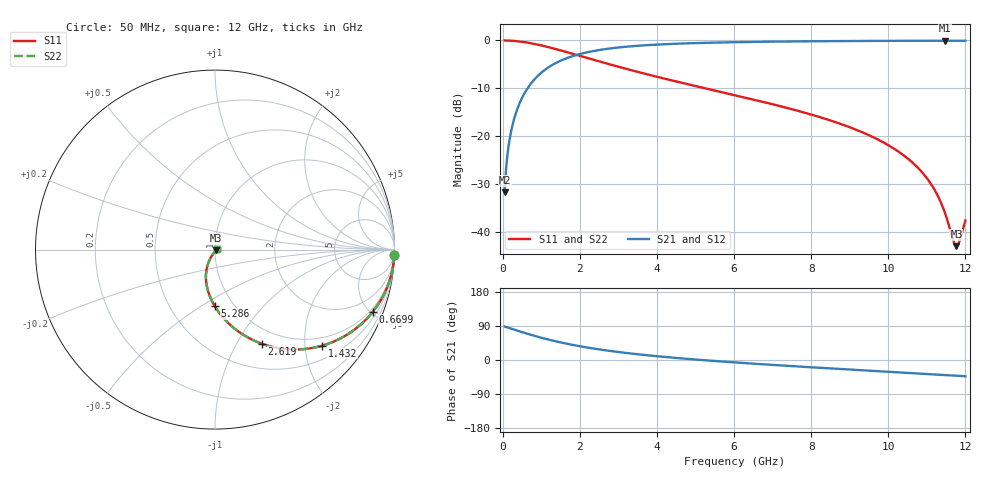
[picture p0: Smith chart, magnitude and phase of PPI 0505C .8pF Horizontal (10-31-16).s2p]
# MHz S MA R 50
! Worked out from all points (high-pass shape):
!   1601 points, 50 MHz to 12 GHz, reference 50 ohm
!   highest |S21| = -0.07 dB at 11.47 GHz (marker M1); lowest = -31.8 dB at 50 MHz (marker M2)
!   |S21| within 3 dB of the highest: 1.899 GHz to end of sweep
!   lowest |S11| = -43.0 dB at 11.77 GHz (marker M3), VSWR 1.01, Z = 50.5 - j0.486 ohm
!   |S11| at or under -10 dB: 5.255 GHz to end of sweep
!   |S22| runs from -43.0 to 0.0 dB; largest |S21 - S12| = 0
!   S11 on the Smith chart (normalised r, x): 50 MHz: 1, -69; 669.9 MHz: 0.79, -5.13; 1.432 GHz: 0.80, -2.38; 2.619 GHz: 0.80, -1.28; 5.286 GHz: 0.82, -0.57; 12 GHz: 1.03, +0.01
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50  0.9997 -1.7  0.02582 88.3  0.02582 88.3  0.9997 -1.7
162.0312  0.9965 -5.4  0.08342 84.6  0.08342 84.6  0.9965 -5.4
266.5938  0.9906 -8.8  0.1365 81.2  0.1365 81.2  0.9906 -8.8
438.375  0.9752 -14.4  0.221 75.6  0.221 75.6  0.9752 -14.4
669.9062  0.9447 -21.6  0.3273 68.4  0.3273 68.4  0.9447 -21.6
1006  0.8864 -31.2  0.4618 58.7  0.4618 58.7  0.8864 -31.2
1431.719  0.8018 -41.9  0.596 48.0  0.596 48.0  0.8018 -41.9
2044.156  0.6826 -54.3  0.7286 35.5  0.7286 35.5  0.6826 -54.3
2619.25  0.5861 -63.5  0.8076 26.2  0.8076 26.2  0.5861 -63.5
4038.312  0.414 -79.9  0.9068 9.6  0.9068 9.6  0.414 -79.9
5285.594  0.3142 -90.3  0.9452 -1.0  0.9452 -1.0  0.3142 -90.3
6025  0.2679 -95.5  0.9589 -6.4  0.9589 -6.4  0.2679 -95.5
8019.156  0.1675 -107.6  0.9803 -19.3  0.9803 -19.3  0.1675 -107.6
9154.406  0.1174 -113.4  0.9869 -26.1  0.9869 -26.1  0.1174 -113.4
10013.31  0.08006 -116.8  0.9901 -31.2  0.9901 -31.2  0.08006 -116.8
10917.03  0.04019 -117.0  0.992 -36.5  0.992 -36.5  0.04019 -117.0
11230.72  0.02621 -113.4  0.9922 -38.3  0.9922 -38.3  0.02621 -113.4
11469.72  0.01582 -103.8  0.9923 -39.7  0.9923 -39.7  0.01582 -103.8
11686.31  0.008127 -70.9  0.9922 -41.0  0.9922 -41.0  0.008127 -70.9
11768.47  0.007103 -42.6  0.9922 -41.5  0.9922 -41.5  0.007103 -42.6
11835.69  0.007777 -18.7  0.9921 -41.9  0.9921 -41.9  0.007777 -18.7
12000  0.01316 13.7  0.992 -42.9  0.992 -42.9  0.01316 13.7
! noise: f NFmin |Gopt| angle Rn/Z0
50  0.001326  0.975  1.386  0.01204
1372  0.005842  0.7727  7.856  0.005221
2701  0.009156  0.7185  12.21  0.006364
4031  0.0121  0.6877  16.68  0.007372
5360  0.01486  0.6678  21.15  0.008311
6682  0.01754  0.6549  25.54  0.00923
8012  0.02023  0.6469  29.88  0.01017
9341  0.02296  0.643  34.11  0.01117
1.067e+04  0.02578  0.6425  38.22  0.01225
1.2e+04  0.02874  0.645  42.22  0.01344
